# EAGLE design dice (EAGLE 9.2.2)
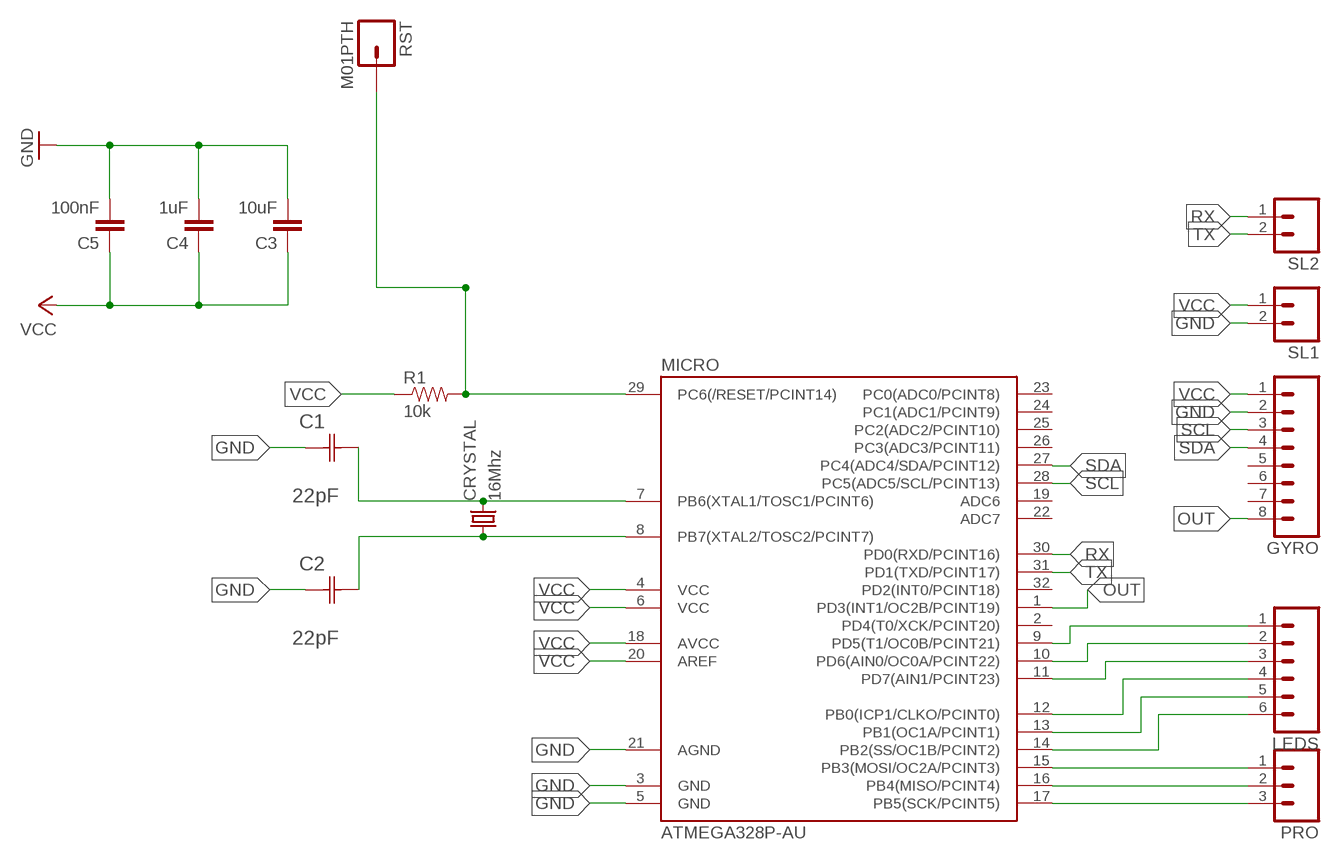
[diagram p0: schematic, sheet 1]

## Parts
C1  22pF  0612ZC225MAT2A  [CAPC3216X178N]
C2  22pF  0612ZC225MAT2A  [CAPC3216X178N]
C3  10uF  CAP1206  [1206]
C4  1uF  CAP1206  [1206]
C5  100nF  CAP1206  [1206]
CRYSTAL  16Mhz  CSM-7X-DU  [CSM-7X-DU]
GYRO  M08  [08P]
LEDS  M06  [06P]
MICRO  ATMEGA328P-AU  ATMEGA48/88/168-AU  [TQFP32-08]
PRO  M03  [03P]
R1  10k  RESISTOR1206  [1206]
RST  M01PTH  [1X01]
SL1  M02  [02P]
SL2  M02  [02P]

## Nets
GND: C1.1(C1) C2.1(C1) C3.2 C4.2 C5.2 GYRO.2 MICRO.3(GND) MICRO.5(GND) MICRO.21(AGND) SL1.2
N$1: MICRO.15(PB3(MOSI/OC2A/PCINT3)) PRO.1
N$2: C1.2(C2) CRYSTAL.2 MICRO.7(PB6(XTAL1/TOSC1/PCINT6))
N$3: MICRO.16(PB4(MISO/PCINT4)) PRO.2
N$4: MICRO.17(PB5(SCK/PCINT5)) PRO.3
N$5: LEDS.1 MICRO.9(PD5(T1/OC0B/PCINT21))
N$6: LEDS.2 MICRO.10(PD6(AIN0/OC0A/PCINT22))
N$7: LEDS.3 MICRO.11(PD7(AIN1/PCINT23))
N$8: LEDS.4 MICRO.12(PB0(ICP1/CLKO/PCINT0))
N$9: C2.2(C2) CRYSTAL.1 MICRO.8(PB7(XTAL2/TOSC2/PCINT7))
N$10: LEDS.5 MICRO.13(PB1(OC1A/PCINT1))
N$11: LEDS.6 MICRO.14(PB2(SS/OC1B/PCINT2))
N$12: MICRO.29(PC6(/RESET/PCINT14)) R1.2 RST.1
OUT: GYRO.8 MICRO.1(PD3(INT1/OC2B/PCINT19))
RX: MICRO.30(PD0(RXD/PCINT16)) SL2.1
SCL: GYRO.3 MICRO.28(PC5(ADC5/SCL/PCINT13))
SDA: GYRO.4 MICRO.27(PC4(ADC4/SDA/PCINT12))
TX: MICRO.31(PD1(TXD/PCINT17)) SL2.2
VCC: C3.1 C4.1 C5.1 GYRO.1 MICRO.4(VCC) MICRO.6(VCC) MICRO.18(AVCC) MICRO.20(AREF) R1.1 SL1.1
Unconnected: GYRO.5 GYRO.6 GYRO.7 MICRO.2(PD4(T0/XCK/PCINT20)) MICRO.19(ADC6) MICRO.22(ADC7) MICRO.23(PC0(ADC0/PCINT8)) MICRO.24(PC1(ADC1/PCINT9)) MICRO.25(PC2(ADC2/PCINT10)) MICRO.26(PC3(ADC3/PCINT11)) MICRO.32(PD2(INT0/PCINT18))

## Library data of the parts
C1 C2 = AVX_By_element14_Batch_1:0612ZC225MAT2A: Capacitor 1206; MPN: 0612ZC225MAT2A; OC_FARNELL: -; OC_NEWARK: 12N3209; SUPPLIER: AVX; TOLERANCE: ±20%; VALUE: 2.2µF; VOLTAGERATING: 10V
C3-C5 = 01_SparkFun:CAP: Capacitor
CRYSTAL = 01_FAB_Hello:CSM-7X-DU: SMD CRYSTAL; OC_FARNELL: unknown; OC_NEWARK: unknown
GYRO = con-amp-quick:M08: AMP QUICK CONNECTOR; OC_FARNELL: unknown; OC_NEWARK: unknown
LEDS = con-amp-quick:M06: AMP QUICK CONNECTOR; OC_FARNELL: unknown; OC_NEWARK: unknown
MICRO = atmega8:ATMEGA48/88/168
PRO = con-amp-quick:M03: AMP QUICK CONNECTOR; OC_FARNELL: unknown; OC_NEWARK: unknown
R1 = 01_SparkFun:RESISTOR: Resistor
RST = 01_SparkFun:M01: Header 1
SL1 SL2 = con-amp-quick:M02: AMP QUICK CONNECTOR; OC_FARNELL: unknown; OC_NEWARK: unknown

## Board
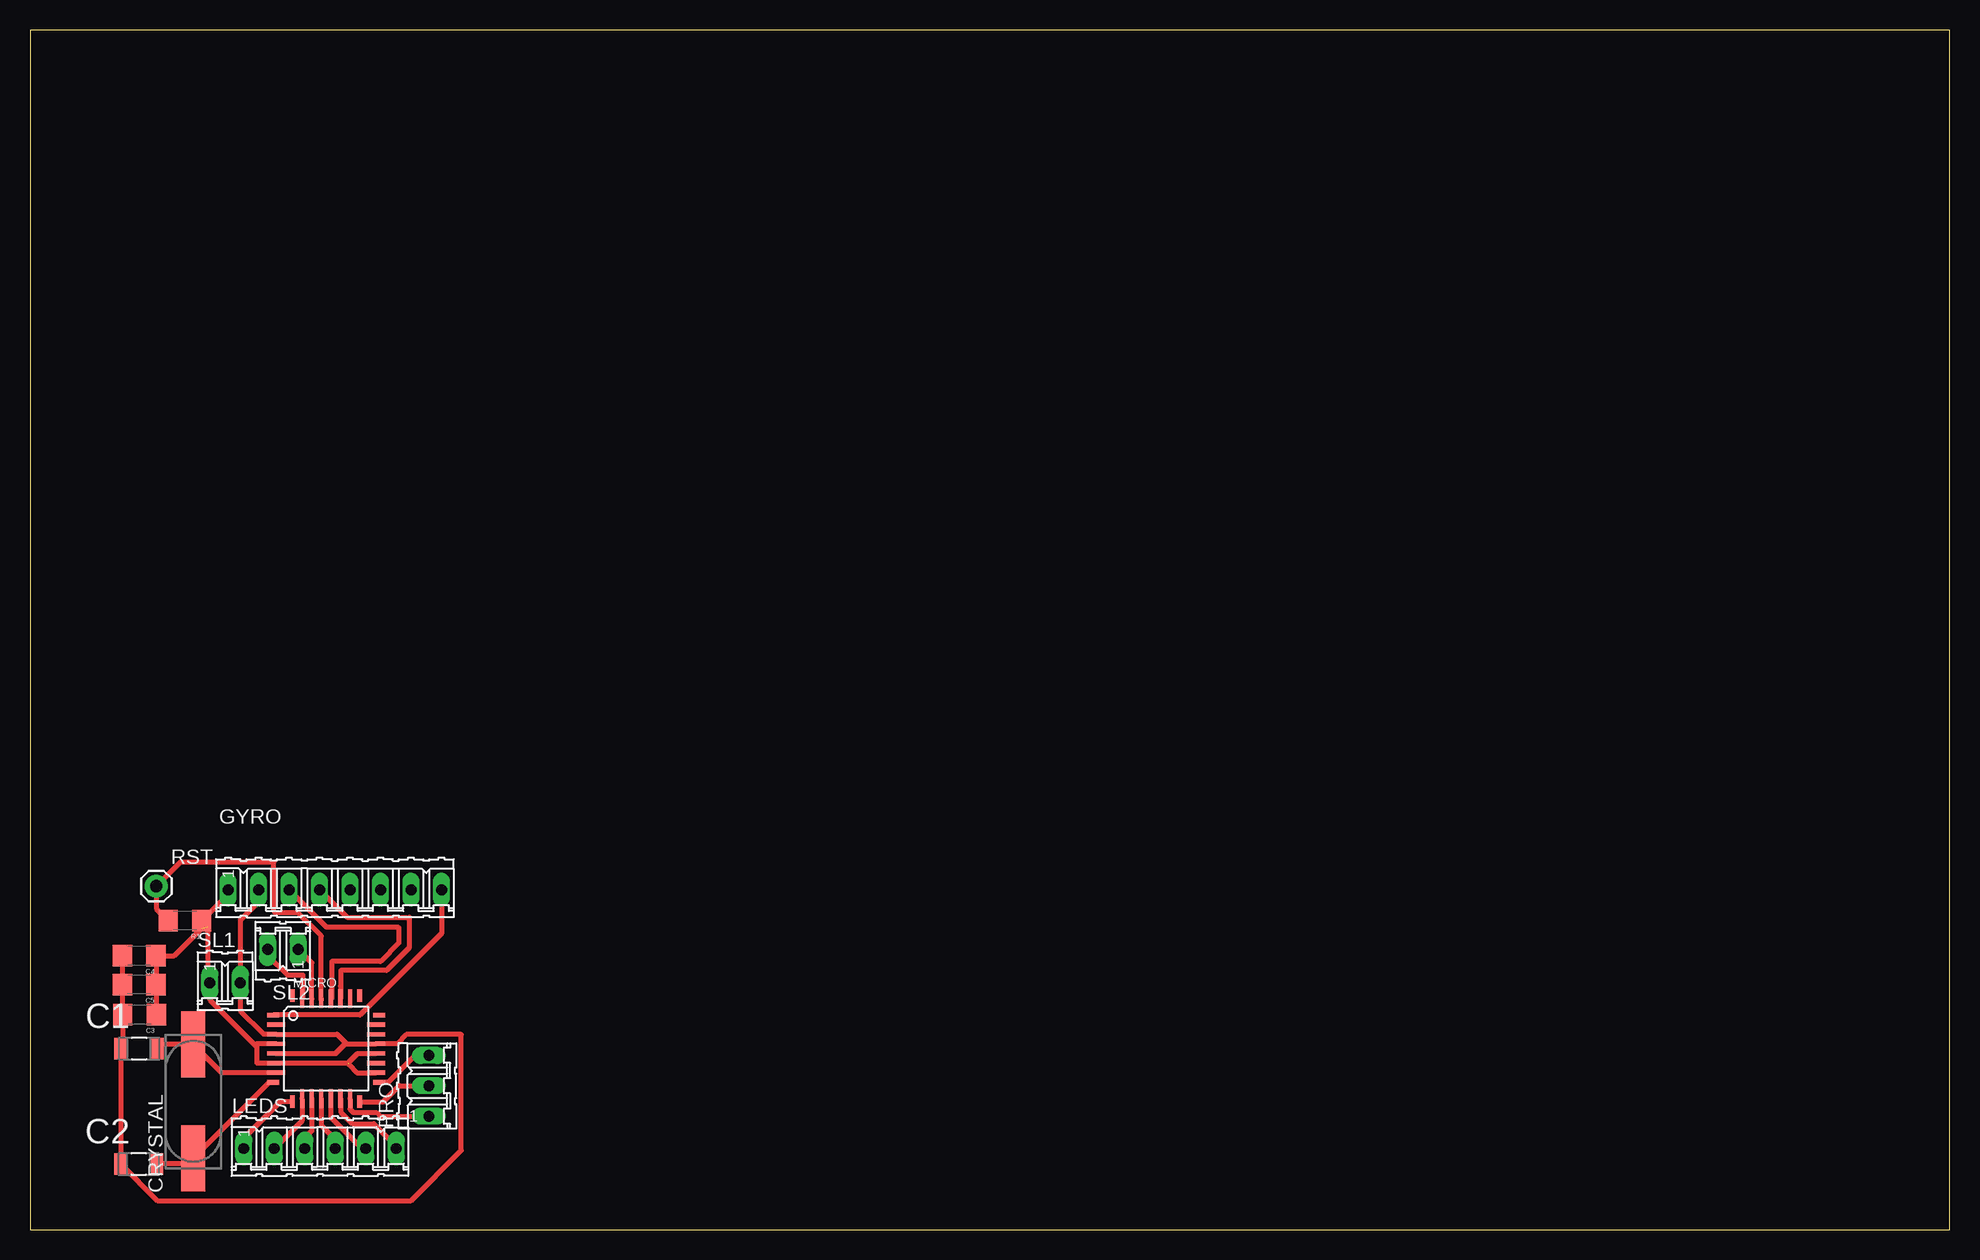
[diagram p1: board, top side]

Size 160 x 100 mm. Coordinates in mm from the lower left corner, seen from the top.
Outline: 0,0 160,0 160,100 0,100 0,0
Copper layers (1*16): Top 0.035mm / dielectric 1.5mm / Bottom 0.035mm
Design rules "default": minimum track width 6mil, minimum drill 0.35mm, track to track 6mil, track to pad 6mil, pad to pad 6mil, via to via 6mil, smd to smd 6mil, copper to edge 40mil, drill to drill 6mil, minimum pad ring 10mil, minimum via ring 8mil, stop-mask expansion 4mil, vias tented up to drill 0mil, thermal gap 10mil

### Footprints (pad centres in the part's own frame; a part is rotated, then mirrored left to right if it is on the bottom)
CAPC3216X178N = smd 1.118 x 1.803: 1 -1.499,0; 2 1.499,0
1206 = smd 1.6 x 1.8: 1 -1.4,0; 2 1.4,0
CSM-7X-DU = smd 5.5 x 2: 1 -4.75,0; 2 4.75,0
08P = drill 0.914 long: 1 -8.89,0; 2 -6.35,0; 3 -3.81,0; 4 -1.27,0; 5 1.27,0; 6 3.81,0; 7 6.35,0; 8 8.89,0
06P = drill 0.914 long: 1 -6.35,0; 2 -3.81,0; 3 -1.27,0; 4 1.27,0; 5 3.81,0; 6 6.35,0
TQFP32-08 = smd 1.016 x 0.406: 1 -4.42,2.8; 8 -4.42,-2.8; 17 4.42,-2.8; 24 4.42,2.8 | smd 1.524 x 0.356: 2 -4.166,2; 3 -4.166,1.2; 4 -4.166,0.4; 5 -4.166,-0.4; 6 -4.166,-1.2; 7 -4.166,-2; 18 4.166,-2; 19 4.166,-1.2; 20 4.166,-0.4; 21 4.166,0.4; 22 4.166,1.2; 23 4.166,2 | smd 0.406 x 1.016: 9 -2.8,-4.42; 16 2.8,-4.42; 25 2.8,4.42; 32 -2.8,4.42 | smd 0.356 x 1.524: 10 -2,-4.166; 11 -1.2,-4.166; 12 -0.4,-4.166; 13 0.4,-4.166; 14 1.2,-4.166; 15 2,-4.166; 26 2,4.166; 27 1.2,4.166; 28 0.4,4.166; 29 -0.4,4.166; 30 -1.2,4.166; 31 -2,4.166
03P = drill 0.914 long: 1 -2.54,0; 2 0,0; 3 2.54,0
1X01 = drill 1.016 pad 1.88: 1 0,0
02P = drill 0.914 long: 1 -1.27,0; 2 1.27,0

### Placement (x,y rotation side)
C1  9.09,15.08 0 top
C2  9.06,5.46 0 top
C3  9.13,17.91 180 top
C4  9.1,22.83 180 top
C5  9.1,20.41 180 top
CRYSTAL  13.62,10.7 90 top
GYRO  25.41,28.32 0 top
LEDS  24.17,6.75 0 top
MICRO  24.68,15.08 0 top
PRO  33.25,11.98 90 top
R1  12.91,25.75 180 top
RST  10.52,28.62 0 top
SL1  16.26,20.57 0 top
SL2  21.08,23.37 180 top

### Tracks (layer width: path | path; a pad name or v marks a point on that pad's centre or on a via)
GND
  Top 0.406: 26.39,15.48 25.59,16.28 MICRO.3 20.5,16.29 19.48,16.29 17.53,18.25 SL1.2 17.54,20.58 17.54,25.78 19.06,27.3 GYRO.2 | 26.39,15.48 26.29,15.48 25.49,14.68 MICRO.5 | 26.39,15.48 MICRO.21 30.59,15.48 31.37,16.26 35.94,16.26 35.94,6.6 31.75,2.41 10.61,2.41 C2.1 7.56,15.05 C1.1 7.74,15.22 C3.2 | 7.7,17.87 C3.2 | 7.7,17.94 C3.2 | C4.2 C5.2 7.7,17.87 | 7.7,17.87 7.59,17.77
N$1
  Top 0.406: MICRO.15 26.68,10.02 26.95,9.75 28.88,9.75 29.19,9.44 PRO.1
N$2
  Top 0.406: MICRO.7 15.98,13.08 CRYSTAL.2 10.96,15.45 C1.2
N$3
  Top 0.406: MICRO.16 29.46,10.66 30.78,11.98 PRO.2
N$4
  Top 0.406: MICRO.17 29.11,12.29 29.88,12.29 32.11,14.52 PRO.3
N$5
  Top 0.406: MICRO.9 20.86,10.66 17.82,7.62 LEDS.1
N$6
  Top 0.406: MICRO.10 22.68,9.07 LEDS.2
N$7
  Top 0.406: MICRO.11 23.48,8.22 22.9,7.64 LEDS.3
N$8
  Top 0.406: MICRO.12 24.28,8.67 25.44,7.51 LEDS.4
N$9
  Top 0.406: MICRO.8 19.95,12.28 CRYSTAL.1 13.13,5.46 C2.2
N$10
  Top 0.406: MICRO.13 25.08,9.34 27.67,6.75 LEDS.5
N$11
  Top 0.406: 25.89,10.9 MICRO.14 25.91,10.89 25.91,9.78 26.87,8.81 28.65,8.81 30.52,6.94 LEDS.6
N$12
  Top 0.406: 24.28,19.12 MICRO.29 24.28,24.46 22.32,26.42 20.45,26.42 20.32,26.54 20.32,30.61 12.51,30.61 RST.1 10.52,26.74 R1.2
OUT
  Top 0.406: GYRO.8 34.3,24.67 27.5,17.88 MICRO.1
RX
  Top 0.406: MICRO.30 23.48,22.24 SL2.1
SCL
  Top 0.406: GYRO.3 24.7,25.21 30.67,25.21 30.73,25.15 30.73,23.88 29.21,22.35 25.15,22.35 25.15,19.31 MICRO.28
SDA
  Top 0.406: GYRO.4 26.43,26.04 31.62,26.04 31.62,23.5 29.72,21.59 25.91,21.59 25.91,20.32 25.88,20.29 MICRO.27
TX
  Top 0.406: SL2.2 19.81,22.86 21.46,21.21 22.73,21.21 22.73,19.3 MICRO.31
VCC  (2 unrouted)
  Top 0.406: MICRO.4 18.91,15.48 18.91,15.24 | MICRO.20 28.83,14.67 27.3,14.67 26.51,13.88 MICRO.6 18.91,13.88 18.91,15.24 | 26.54,13.75 27.22,13.08 MICRO.18 | 14.99,20.58 SL1.1 | SL1.1 14.99,19.16 18.91,15.24 | 10.5,20.7 C4.1 12.03,22.83 14.31,25.11 | 10.5,20.7 C5.1 10.5,17.94 C3.1 | 10.54,20.67 10.5,20.7 | GYRO.1 16.52,27.95 R1.1 14.82,25.24 14.82,20.74 SL1.1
